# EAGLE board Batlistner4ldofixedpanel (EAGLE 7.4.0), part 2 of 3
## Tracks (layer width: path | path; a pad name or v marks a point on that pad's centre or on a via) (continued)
GND  (via drill 0.5) (continued)
  Top 0.406: IC1.3 15.24,18.73 15.88,17.78 15.88,17.24 C8.2 | 12.06,34.61 v11.75,34.92 12.38,34.29 C16.2 12.97,33.66 C4.2 | IC3.2 41.27,11.74 C13.1 | R12.1 32.06,20.64 v31.11,19.68 30.32,19.05 | v18.41,36.51 18.41,36.2 19.37,35.24 | v23.02,4.29 23.02,3.81 22.7,3.49
  Bottom 0.254: 45.75,9 46.04,8.89 | 9,31.5 SG1.- 8.75,31.75
  other vias: 17.78,12.06 24.13,20.95 12.06,22.23 9.21,27.94 14.29,1.27 31.75,31.11 11.43,38.73 10.16,49.21 34.29,34.92 23.5,30.16 41.91,34.92 44.45,34.92 46.67,39.69 37.78,25.72 20,42.55 1.91,54.61 9.53,54.61 17.14,54.61 22.23,54.61 10.16,46.35 10.16,43.81 1.91,38.73 9.53,1.27 18.1,25.72 24.13,16.67 40.01,1.27 47.62,1.27 60.33,1.27 62.87,6.35 62.87,13.97 62.87,21.59 62.87,33.02 62.87,40.64 62.87,48.26 31.11,54.61 31.91,25.72 40.01,16.51 46.35,20.32 45.88,10.32 53.66,26.04 49.21,29.84 41.91,47.94 38.1,39.37 36.83,42.86 1.91,45.72 14.29,13.02 14.29,7.94 10.17,41.35 21.27,46.99 56.52,43.18
  pour Top: 6.99,-0.64 7.62,19.05 7.94,22.86 7.62,24.77 8.26,35.56 6.99,36.83 0,36.83 0,55.88 64.14,55.88 64.14,31.75 62.23,27.94 64.77,24.13 64.14,0
  pour Bottom: 64.14,0 6.99,-0.64 7.62,15.24 7.62,20 8.26,20.32 8.26,35.56 6.35,37.47 0,36.83 0,55.88 64.77,55.88 64.77,31.75 62.23,27.94 64.77,24.13
GND1  (via drill 0.5)
  Top 0.406: IC7.3 83.82,18.73 84.45,17.78 84.45,17.24 C55.2 | 80.64,34.61 v80.33,34.92 80.96,34.29 C58.2 81.55,33.66 C57.2 | IC9.2 109.86,11.74 C49.1 | R43.1 100.64,20.64 v99.69,19.68 98.9,19.05 | v87,36.51 87,36.2 87.95,35.24 | v91.6,4.29 91.6,3.81 91.28,3.49
  Bottom 0.254: 114.33,9 114.62,8.89 | 77.58,31.5 SG3.- 77.33,31.75
  other vias: 86.36,12.06 92.71,20.95 80.64,22.23 77.79,27.94 82.87,1.27 100.33,31.11 80.01,38.73 78.74,49.21 102.87,34.92 92.08,30.16 110.49,34.92 113.03,34.92 115.25,39.69 106.36,25.72 88.58,42.55 70.48,54.61 78.11,54.61 85.72,54.61 90.81,54.61 78.74,46.35 78.74,43.81 70.48,38.73 78.11,1.27 86.68,25.72 92.71,16.67 108.58,1.27 116.2,1.27 128.91,1.27 131.44,6.35 131.44,13.97 131.44,21.59 131.44,33.02 131.44,40.64 131.44,48.26 99.69,54.61 100.49,25.72 108.58,16.51 114.94,20.32 114.46,10.32 122.24,26.04 117.79,29.84 110.49,47.94 106.68,39.37 105.41,42.86 70.48,45.72 82.87,13.02 82.87,7.94 78.75,41.35 89.85,46.99 125.09,43.18
  pour Top: 75.56,-0.64 76.2,19.05 76.52,22.86 76.2,24.77 76.83,35.56 75.56,36.83 68.58,36.83 68.58,55.88 132.72,55.88 132.72,31.75 130.81,27.94 133.35,24.13 132.72,0
  pour Bottom: 132.72,0 75.56,-0.64 76.2,15.24 76.2,20 76.83,20.32 76.83,35.56 74.93,37.47 68.58,36.83 68.58,55.88 133.35,55.88 133.35,31.75 130.81,27.94 133.35,24.13
GND2  (via drill 0.5)
  Top 0.406: IC13.3 152.4,18.73 153.03,17.78 153.03,17.24 C100.2 | 149.22,34.61 v148.91,34.92 149.54,34.29 C103.2 150.13,33.66 C102.2 | IC15.2 178.44,11.74 C94.1 | R82.1 169.22,20.64 v168.28,19.68 167.48,19.05 | v155.57,36.51 155.57,36.2 156.53,35.24 | v160.18,4.29 160.18,3.81 159.86,3.49
  Bottom 0.254: 182.91,9 183.2,8.89 | 146.16,31.5 SG5.- 145.91,31.75
  other vias: 154.94,12.06 161.29,20.95 149.22,22.23 146.37,27.94 151.45,1.27 168.91,31.11 148.59,38.73 147.32,49.21 171.45,34.92 160.66,30.16 179.07,34.92 181.61,34.92 183.83,39.69 174.94,25.72 157.16,42.55 139.06,54.61 146.69,54.61 154.31,54.61 159.38,54.61 147.32,46.35 147.32,43.81 139.06,38.73 146.69,1.27 155.26,25.72 161.29,16.67 177.16,1.27 184.78,1.27 197.49,1.27 200.03,6.35 200.03,13.97 200.03,21.59 200.03,33.02 200.03,40.64 200.03,48.26 168.28,54.61 169.07,25.72 177.16,16.51 183.51,20.32 183.04,10.32 190.82,26.04 186.37,29.84 179.07,47.94 175.26,39.37 173.99,42.86 139.06,45.72 151.45,13.02 151.45,7.94 147.33,41.35 158.43,46.99 193.68,43.18
  pour Top: 144.15,-0.64 144.78,19.05 145.1,22.86 144.78,24.77 145.41,35.56 144.15,36.83 137.16,36.83 137.16,55.88 201.29,55.88 201.29,31.75 199.39,27.94 201.93,24.13 201.29,0
  pour Bottom: 201.29,0 144.15,-0.64 144.78,15.24 144.78,20 145.41,20.32 145.41,35.56 143.51,37.47 137.16,36.83 137.16,55.88 201.93,55.88 201.93,31.75 199.39,27.94 201.93,24.13
GND3  (via drill 0.5)
  Top 0.406: IC19.3 15.24,79.69 15.88,78.74 15.88,78.2 C145.2 | 12.06,95.57 v11.75,95.89 12.38,95.25 C148.2 12.97,94.61 C147.2 | IC21.2 41.27,72.7 C139.1 | R121.1 32.06,81.59 v31.11,80.64 30.32,80.01 | v18.41,97.47 18.41,97.16 19.37,96.2 | v23.02,65.25 23.02,64.77 22.7,64.45
  Bottom 0.254: 45.75,69.96 46.04,69.85 | 9,92.46 SG7.- 8.75,92.71
  other vias: 17.78,73.03 24.13,81.92 12.06,83.19 9.21,88.9 14.29,62.23 31.75,92.08 11.43,99.69 10.16,110.17 34.29,95.89 23.5,91.12 41.91,95.89 44.45,95.89 46.67,100.65 37.78,86.68 20,103.5 1.91,115.57 9.53,115.57 17.14,115.57 22.23,115.57 10.16,107.31 10.16,104.78 1.91,99.69 9.53,62.23 18.1,86.68 24.13,77.63 40.01,62.23 47.62,62.23 60.33,62.23 62.87,67.31 62.87,74.93 62.87,82.55 62.87,93.98 62.87,101.6 62.87,109.22 31.11,115.57 31.91,86.68 40.01,77.47 46.35,81.28 45.88,71.28 53.66,87 49.21,90.81 41.91,108.9 38.1,100.33 36.83,103.82 1.91,106.68 14.29,73.98 14.29,68.9 10.17,102.31 21.27,107.95 56.52,104.14
  pour Top: 6.99,60.33 7.62,80.01 7.94,83.82 7.62,85.72 8.26,96.52 6.99,97.79 0,97.79 0,116.84 64.14,116.84 64.14,92.71 62.23,88.9 64.77,85.09 64.14,60.96
  pour Bottom: 64.14,60.96 6.99,60.33 7.62,76.2 7.62,80.96 8.26,81.28 8.26,96.52 6.35,98.42 0,97.79 0,116.84 64.77,116.84 64.77,92.71 62.23,88.9 64.77,85.09
GND4  (via drill 0.5)
  Top 0.406: IC25.3 83.82,79.69 84.45,78.74 84.45,78.2 C190.2 | 80.64,95.57 v80.33,95.89 80.96,95.25 C193.2 81.55,94.61 C192.2 | IC27.2 109.86,72.7 C184.1 | R160.1 100.64,81.59 v99.69,80.64 98.9,80.01 | v87,97.47 87,97.16 87.95,96.2 | v91.6,65.25 91.6,64.77 91.28,64.45
  Bottom 0.254: 114.33,69.96 114.62,69.85 | 77.58,92.46 SG9.- 77.33,92.71
  other vias: 86.36,73.03 92.71,81.92 80.64,83.19 77.79,88.9 82.87,62.23 100.33,92.08 80.01,99.69 78.74,110.17 102.87,95.89 92.08,91.12 110.49,95.89 113.03,95.89 115.25,100.65 106.36,86.68 88.58,103.5 70.48,115.57 78.11,115.57 85.72,115.57 90.81,115.57 78.74,107.31 78.74,104.78 70.48,99.69 78.11,62.23 86.68,86.68 92.71,77.63 108.58,62.23 116.2,62.23 128.91,62.23 131.44,67.31 131.44,74.93 131.44,82.55 131.44,93.98 131.44,101.6 131.44,109.22 99.69,115.57 100.49,86.68 108.58,77.47 114.94,81.28 114.46,71.28 122.24,87 117.79,90.81 110.49,108.9 106.68,100.33 105.41,103.82 70.48,106.68 82.87,73.98 82.87,68.9 78.75,102.31 89.85,107.95 125.09,104.14
  pour Top: 75.56,60.33 76.2,80.01 76.52,83.82 76.2,85.72 76.83,96.52 75.56,97.79 68.58,97.79 68.58,116.84 132.72,116.84 132.72,92.71 130.81,88.9 133.35,85.09 132.72,60.96
  pour Bottom: 132.72,60.96 75.56,60.33 76.2,76.2 76.2,80.96 76.83,81.28 76.83,96.52 74.93,98.42 68.58,97.79 68.58,116.84 133.35,116.84 133.35,92.71 130.81,88.9 133.35,85.09
GND5  (via drill 0.5)
  Top 0.406: IC31.3 152.4,79.69 153.03,78.74 153.03,78.2 C235.2 | 149.22,95.57 v148.91,95.89 149.54,95.25 C238.2 150.13,94.61 C237.2 | IC33.2 178.44,72.7 C229.1 | R199.1 169.22,81.59 v168.28,80.64 167.48,80.01 | v155.57,97.47 155.57,97.16 156.53,96.2 | v160.18,65.25 160.18,64.77 159.86,64.45
  Bottom 0.254: 182.91,69.96 183.2,69.85 | 146.16,92.46 SG11.- 145.91,92.71
  other vias: 154.94,73.03 161.29,81.92 149.22,83.19 146.37,88.9 151.45,62.23 168.91,92.08 148.59,99.69 147.32,110.17 171.45,95.89 160.66,91.12 179.07,95.89 181.61,95.89 183.83,100.65 174.94,86.68 157.16,103.5 139.06,115.57 146.69,115.57 154.31,115.57 159.38,115.57 147.32,107.31 147.32,104.78 139.06,99.69 146.69,62.23 155.26,86.68 161.29,77.63 177.16,62.23 184.78,62.23 197.49,62.23 200.03,67.31 200.03,74.93 200.03,82.55 200.03,93.98 200.03,101.6 200.03,109.22 168.28,115.57 169.07,86.68 177.16,77.47 183.51,81.28 183.04,71.28 190.82,87 186.37,90.81 179.07,108.9 175.26,100.33 173.99,103.82 139.06,106.68 151.45,73.98 151.45,68.9 147.33,102.31 158.43,107.95 193.68,104.14
  pour Top: 144.15,60.33 144.78,80.01 145.1,83.82 144.78,85.72 145.41,96.52 144.15,97.79 137.16,97.79 137.16,116.84 201.29,116.84 201.29,92.71 199.39,88.9 201.93,85.09 201.29,60.96
  pour Bottom: 201.29,60.96 144.15,60.33 144.78,76.2 144.78,80.96 145.41,81.28 145.41,96.52 143.51,98.42 137.16,97.79 137.16,116.84 201.93,116.84 201.93,92.71 199.39,88.9 201.93,85.09
N$1  (1 unrouted)
  Top 0.406: C36.2 C35.2 C34.2 C33.2 | C37.2 C38.2 C39.2 C40.2 C3.2 52.7,13.81 | 52.7,13.81 52.71,13.81 C32.2 | 52.7,13.81 52.7,13.34 48.74,13.34 47.78,12.38 47.78,10 48.26,9.53 49.66,9.53 U$1.P$4 50.3,9.39 53.98,5.71 56.66,5.71 U$1.P$3
N$2
  Top 0.406: C14.1 46.35,6.67 R14.1
N$3
  Top 0.254: Q1.C 20.64,1.91 20.32,1.59
  Top 0.406: R5.1 20.32,1.59 C7.1 | R4.2 Q1.C
N$4
  Top 0.406: IC3.7 41.27,17.78 41.91,17.14 44.77,17.14 C15.2
N$5
  Top 0.406: IC1.4 16.51,19.68 18.41,17.78 18.73,17.78 R8.1
N$6
  Top 0.406: R8.2 C9.1
N$7  (1 unrouted)
  Top 0.406: C81.2 C80.2 C79.2 C78.2 | C82.2 C83.2 C84.2 C85.2 C76.2 121.28,13.81 | 121.28,13.81 121.29,13.81 C77.2 | 121.28,13.81 121.28,13.34 117.32,13.34 116.36,12.38 116.36,10 116.84,9.53 118.23,9.53 U$2.P$4 118.88,9.39 122.56,5.71 125.25,5.71 U$2.P$3
N$8
  Top 0.406: IC2.3 27.94,18.41 32.7,18.41 R12.2 34.75,18.73 R13.2 36.66,18.56 R11.1
N$9
  Top 0.406: S1.3 49.39,50.94 50.16,50.16 53.34,50.16 54.61,48.9 D1.A 55.49,47.62 C45.1 C44.1
N$10
  Top 0.406: SG1.+ 9.21,23.81 10.16,22.86 C5.2
N$11
  Top 0.406: 12.06,15.72 Q2.B 11.91,15.88 11.11,15.88 10.79,16.2 R1.1 9.84,15.88 8.89,17.14 8.89,19.37 9.53,20 C5.1
N$12
  Top 0.254: 14.44,15.09 13.02,16.51 11.75,16.51
  Top 0.406: R36.2 14.93,6.67 C6.2 15.88,8.57 16.83,9.53 16.83,10.62 Q3.C 16.66,13.51 R2.2 15.38,13.65 Q2.C 14.44,15.09 | 11.75,16.51 11.43,16.83 11.43,17.78 11.11,18.1 R1.2
N$13
  Top 0.406: 22.22,15.24 R3.2 | C26.1 C25.1 C24.1 C2.1 22.23,12.7 | 22.23,12.7 R3.2 | R2.1 17.14,15.56 R3.2 | R3.2 | 20.95,10.16 R4.1 21.27,9.84 22.23,10.79 22.23,12.7 | 20.95,11.43 22.23,12.7
N$14
  Top 0.406: C7.2 22.86,2.54 24.13,3.81 24.13,5.88 R7.1
N$15
  Top 0.406: R10.1 31.43,11.72 R17.P$1
N$16
  Top 0.406: R6.1 18.1,3.81 | R5.2 17.46,3.81 R6.1 | Q1.B 18.25,3.66 R6.1
N$17
  Top 0.406: C6.1 R6.2
N$18  (via drill 0.5)
  Top 0.406: IC1.1 v12.7,17.78 | v25.72,9.21 23.5,9.21 R7.2
  Bottom 0.406: v12.7,17.78 14.61,17.78 v25.72,9.21
N$19
  Top 0.406: C8.1 14.29,18.09 13.97,18.41 IC1.2
N$20  (via drill 0.5)
  Top 0.406: v21.59,24.13 19.37,24.13 C9.2
  Bottom 0.406: R18.P$3 37.34,44.57 40.01,41.91 40.01,32.38 31.75,24.13 v21.59,24.13
N$21
  Top 0.406: C50.1 114.93,6.67 R45.1
N$22  (via drill 0.5)
  Top 0.406: v43.18,8.89 43.18,12.38 C13.2 42.86,13.65 42.55,13.97 IC3.3
  Bottom 0.406: R18.P$1 31.23,44.57 33.02,46.35 37.47,46.35 43.18,40.64 v43.18,8.89
N$23
  Top 0.406: IC4.9 31.43,26.99 31.75,26.67 33.97,26.67 34.61,27.3 34.61,30.16 R29.2 35.88,30.48 36.83,30.48 36.52,30.16 R31.1 36.88,30.11 C22.2
N$24  (via drill 0.5)  (1 unrouted)
  Top 0.406: IC4.19 v22.54,36.2 | v16.83,48.9 16.83,49.21 17.46,49.85 17.46,51.12
  Bottom 0.406: SCK.TP 22.86,36.2 v22.54,36.2 20.64,36.2 16.83,40.01 v16.83,48.9
N$25  (via drill 0.5)  (1 unrouted)
  Top 0.406: R19.1 v18.73,48.89 | v23.5,39.69 23.81,39.37 IC4.18
  Bottom 0.406: MISO.TP 27.3,36.2 25.4,38.1 23.5,38.1 | 23.5,38.1 20.32,38.1 17.78,40.64 17.78,48.9 v18.73,48.9 | 23.5,38.1 v23.5,39.69
N$26  (via drill 0.5)
  Top 0.406: R20.1 17.46,37.47 17.46,35.88 19.05,34.29 24.45,34.29 25.08,34.92 IC4.17 v25.08,39.37 | v29.84,35.56 29.84,31.11 28.89,30.16 v26.04,30.16
  Bottom 0.406: v25.08,39.37 26.04,39.37 v29.84,35.56 | v26.04,30.16 25.72,30.16 24.77,31.11 MOSI.TP
N$27
  Top 0.406: C23.1 43.18,6.99 C14.2 44.13,7.3 44.45,7.62 44.45,11.43 45.08,12.06 45.09,12.06 47.94,14.92 47.94,19.05 | 47.94,19.05 47.94,22.54 50.16,24.77 52.7,24.77 52.7,23.81 | 52.7,23.81 55.24,23.81 55.56,23.5 55.56,19.05 C36.1 C35.1 C34.1 C33.1 C32.1 | C3.1 C40.1 C39.1 C38.1 C37.1 49.85,23.5 50.16,23.81 52.7,23.81 | IC3.5 47.88,19.11 47.94,19.05
N$28
  Top 0.406: IC2.2 26.67,14.29 C12.2 26.99,11.53 R17.P$3
N$29
  Top 0.406: R21.1 16,36.07 18.41,33.66 25.4,33.66 26.35,34.61 IC4.16
N$30  (via drill 0.5)
  Top 0.406: IC1.6 15.24,23.5 v15.88,22.86 | 35.88,24.29 28.1,24.29 27.3,23.5 24.77,23.5 24.13,22.86 v23.5,22.86 | C11.2 35.88,25.4 35.88,24.29 | 35.88,24.29 C10.2
  Bottom 0.406: v15.88,22.86 v23.5,22.86
N$31
  Top 0.406: R22.1 25.08,41.27 27.62,38.73 IC4.15
N$32
  Top 0.406: C11.1 37.15,27.94 38.42,28.26 R9.2
N$33
  Top 0.406: IC4.14 28.89,39.05 24.57,43.37 R23.1
N$34  (via drill 0.5)
  Top 0.406: R24.1 v20,43.81 | v30.16,39.69 IC4.13
  Bottom 0.406: v20,43.81 24.13,43.81 26.04,41.91 27.94,41.91 v30.16,39.69
N$35  (1 unrouted)
  Top 0.406: IC4.12 31.43,40.96 31.11,41.27 30.96,41.43 30.48,41.91
N$36
  Top 0.406: R15.2 15.56,50.8 IC5.5
N$37
  Top 0.406: IC5.4 15.88,46.35 R19.2
N$38
  Top 0.406: IC5.10 9.53,38.73 10.79,40.01 15.55,40.01 R20.2
N$39
  Top 0.406: IC5.1 13.65,36.39 R21.2
N$40
  Top 0.406: IC5.2 R22.2
N$41
  Top 0.406: IC5.3 14.29,43.81 15.56,45.09 20.83,45.09 R23.2
N$42
  Top 0.406: IC5.8 7.3,43.81 8.57,42.55 15.24,42.55 R24.2
N$43
  Top 0.406: IC5.7 7.94,46.35 9.21,45.09 14.61,45.09 15.24,45.72 21.27,45.72 22.07,44.93 25.56,44.93 25.72,44.77 25.72,43.66 27.78,41.59 R25.2
N$44  (via drill 0.5)
  Top 0.406: v28.26,26.99 R39.2
  Bottom 0.406: IC5.9 7.3,41.27 8.26,40.32 8.26,37.47 10.16,35.56 10.16,34.29 12.06,32.38 12.06,29.84 14.92,26.99 v28.26,26.99
N$45  (via drill 0.5)
  Top 0.406: R40.2 20.48,25.24 18.41,27.3 15.88,27.3 v14.61,28.57
  Bottom 0.406: v14.61,28.57 14.61,33.66 8.89,39.37 8.89,47.62 7.62,48.9 IC5.6
N$46
  Top 0.406: IC4.6 27.62,27.62 25.88,25.88 25.88,25.56 R40.1
N$47
  Top 0.406: C16.1 12.75,31.07 13.34,30.48 14.26,30.48 X1.3 14.32,30.12 16.19,28.26 18.73,28.26 20.32,26.67 25.4,26.67 26.35,27.62 IC4.5
N$48
  Top 0.406: R33.2 42.23,25.98 C21.1
N$49  (via drill 0.5)
  Top 0.406: IC4.20 21.27,39.05 21.59,39.37 v21.59,39.69 C17.2 | v38.1,41.27 39.37,41.27 39.49,41.16 | R29.1 34.92,31.75 v31.75,34.92 | R26.1 40.64,40.01 39.49,41.16 | C18.1 41.27,41.91 | 41.27,41.91 40.24,41.91 39.49,41.16 | 39.49,41.16 | IC6.3 41.27,43.58 41.27,41.91
  Bottom 0.406: v38.1,41.27 33.66,41.27 31.75,39.37 31.75,37.47 | VCC.TP 28.57,31.75 v31.75,34.92 31.75,37.47 | 31.75,37.47 30.48,37.47 26.67,41.27 21.59,41.27 v21.59,39.69
N$50
  Top 0.406: R32.1 39.69,7.94 C23.2
N$51
  Top 0.406: R28.1 47.62,36.2 46.35,37.47 44.34,37.47 C20.1 40.82,37.61 R26.2 40.32,37.46 R27.1
N$52
  Top 0.406: C21.2 42.55,29.7 Q4.B R28.2
N$53
  Top 0.406: Q4.C 39.64,32.38 C22.1 39.37,33.66 38.42,34.61 R27.2
N$54  (via drill 0.5)
  Top 0.406: IC4.1 21.01,28.52 v19.05,30.48
  Bottom 0.406: v19.05,30.48 19.05,33.02 20.32,34.29 RES.TP
N$55
  Top 0.406: C41.1 C19.1 43.81,46.09 | 43.81,46.09 39.85,46.09 IC6.2@1 | R30.2 43.81,48.26 43.81,46.09
N$56
  Top 0.406: IC3.1 38.36,13.91 | 38.36,13.91 R32.2 | 38.36,13.91 38.36,14.55 C43.1
N$57
  Top 0.406: R30.1 R35.2 49.85,47.94 50.8,46.99 C28.1
N$58
  Top 0.406: SG2.+ 9.21,12.7 9.84,12.06 C42.2
N$59  (via drill 0.5)
  Top 0.406: C27.2 R34.1 47.31,25.4 44.13,22.23 v40.64,22.23 | 26.67,19.68 24.13,19.68 22.23,17.78 R3.1 v22.23,20.32 | 26.67,19.68 29.53,19.68 31.11,21.11 31.11,21.59 31.75,22.23 v34.29,22.23 34.92,21.59 R13.1 | IC2.7 26.67,19.68 | IC1.8 12.7,22.86 13.34,22.23 v13.97,22.23
  Bottom 0.406: v34.29,22.23 36.2,24.13 38.73,24.13 v40.64,22.23 | v13.97,22.23 14.61,22.23 15.24,21.59 20.95,21.59 v22.23,20.32
N$60
  Top 0.406: R36.1 C42.1 12.88,10.16 Q3.B
N$61
  Top 0.406: C43.2 R37.1
N$62
  Top 0.406: R37.2 38.41,16.82 40.01,18.41 IC3.8
N$63
  Top 0.406: C4.1 15.88,33.66 15.88,31.75 | 15.88,31.75 15.88,29.84 16.51,29.21 18.73,29.21 20.64,27.3 24.77,27.3 25.08,27.62 IC4.4 | X1.1 15.94,31.82 15.88,31.75
N$64
  Top 0.406: U$1.P$1 59.37,4.26 R38.2
N$65
  Top 0.406: U$1.P$5 50.01,11.28 50.32,11.59 53.17,11.6 53.98,10.79 56.48,10.79 U$1.P$6 57.45,11.1 SP1.+
N$66
  Top 0.406: R39.1 30.16,26.51 28.89,27.78 IC4.7
N$67
  Top 0.406: S1.2 52.53,52.88 55.24,50.16 57.15,50.16 57.78,49.53 60.33,49.53 60.96,48.9 60.96,43.18 G1.+
N$68
  Top 0.406: IC9.7 109.86,17.78 110.49,17.14 113.34,17.14 C51.2
N$69
  Top 0.406: IC7.4 85.09,19.68 87,17.78 87.31,17.78 R54.1
N$70
  Top 0.406: R54.2 C56.1
N$71
  Top 0.406: SG3.+ 77.79,23.81 78.74,22.86 C52.2
N$72
  Top 0.406: 80.64,15.72 Q6.B 80.5,15.88 79.69,15.88 79.37,16.2 R16.1 78.42,15.88 77.47,17.14 77.47,19.37 78.11,20 C52.1
N$73
  Top 0.254: 83.02,15.09 81.6,16.51 80.33,16.51
  Top 0.406: R74.2 83.51,6.67 C53.2 84.46,8.57 85.41,9.53 85.41,10.62 Q8.C 85.24,13.51 R48.2 83.97,13.65 Q6.C 83.02,15.09 | 80.33,16.51 80.01,16.83 80.01,17.78 79.69,18.1 R16.2
N$74
  Top 0.406: 90.8,15.24 R49.2 | C69.1 C68.1 C67.1 C66.1 90.81,12.7 | 90.81,12.7 R49.2 | R48.1 85.72,15.56 R49.2 | R49.2 | 89.53,10.16 R50.1 89.85,9.84 90.81,10.79 90.81,12.7 | 89.53,11.43 90.81,12.7
N$75
  Top 0.406: R52.1 86.68,3.81 | R51.2 86.05,3.81 R52.1 | Q5.B 86.83,3.66 R52.1
N$76
  Top 0.406: C53.1 R52.2
N$77
  Top 0.254: Q5.C 89.22,1.91 88.9,1.59
  Top 0.406: R51.1 88.9,1.59 C54.1 | R50.2 Q5.C
N$78
  Top 0.406: C54.2 91.44,2.54 92.71,3.81 92.71,5.88 R53.1
N$79  (via drill 0.5)
  Top 0.406: IC7.1 v81.28,17.78 | v94.3,9.21 92.08,9.21 R53.2
  Bottom 0.406: v81.28,17.78 83.19,17.78 v94.3,9.21
N$80
  Top 0.406: C55.1 82.87,18.09 82.55,18.41 IC7.2
N$81  (via drill 0.5)
  Top 0.406: v90.17,24.13 87.95,24.13 C56.2
  Bottom 0.406: R47.P$3 105.92,44.57 108.58,41.91 108.58,32.38 100.33,24.13 v90.17,24.13
N$82  (via drill 0.5)
  Top 0.406: v111.76,8.89 111.76,12.38 C49.2 111.44,13.65 111.12,13.97 IC9.3
  Bottom 0.406: R47.P$1 99.81,44.57 101.6,46.35 106.05,46.35 111.76,40.64 v111.76,8.89
N$83
  Top 0.406: C65.1 111.76,6.99 C50.2 112.71,7.3 113.03,7.62 113.03,11.43 113.66,12.06 113.67,12.06 116.52,14.92 116.52,19.05 | 116.52,19.05 116.52,22.54 118.75,24.77 121.28,24.77 121.28,23.81 | 121.28,23.81 123.83,23.81 124.14,23.5 124.14,19.05 C81.1 C80.1 C79.1 C78.1 C77.1 | C76.1 C85.1 C84.1 C83.1 C82.1 118.43,23.5 118.75,23.81 121.28,23.81 | IC9.5 116.46,19.11 116.52,19.05
N$84
  Top 0.406: IC8.3 96.52,18.41 101.28,18.41 R43.2 103.33,18.73 R44.2 105.23,18.56 R42.1
N$85
  Top 0.406: IC8.2 95.25,14.29 C48.2 95.57,11.53 R46.P$3
N$86  (via drill 0.5)
  Top 0.406: IC7.6 83.82,23.5 v84.45,22.86 | 104.46,24.29 96.68,24.29 95.89,23.5 93.34,23.5 92.71,22.86 v92.08,22.86 | C47.2 104.46,25.4 104.46,24.29 | 104.46,24.29 C46.2
  Bottom 0.406: v84.45,22.86 v92.08,22.86
N$87
  Top 0.406: C47.1 105.72,27.94 107,28.26 R55.2
N$88
  Top 0.406: R41.1 100.02,11.72 R46.P$1
N$89  (via drill 0.5)  (1 unrouted)
  Top 0.406: IC10.19 v91.12,36.2 | v85.41,48.9 85.41,49.21 86.04,49.85 86.04,51.12
  Bottom 0.406: SCK1.TP 91.44,36.2 v91.12,36.2 89.22,36.2 85.41,40.01 v85.41,48.9
N$90  (via drill 0.5)  (1 unrouted)
  Top 0.406: R57.1 v87.31,48.89 | v92.08,39.69 92.39,39.37 IC10.18
  Bottom 0.406: MISO1.TP 95.89,36.2 93.98,38.1 92.08,38.1 | 92.08,38.1 88.9,38.1 86.36,40.64 86.36,48.9 v87.31,48.9 | 92.08,38.1 v92.08,39.69
N$91  (via drill 0.5)
  Top 0.406: R58.1 86.04,37.47 86.04,35.88 87.63,34.29 93.03,34.29 93.66,34.92 IC10.17 v93.66,39.37 | v98.42,35.56 98.42,31.11 97.47,30.16 v94.61,30.16
  Bottom 0.406: v93.66,39.37 94.61,39.37 v98.42,35.56 | v94.61,30.16 94.3,30.16 93.34,31.11 MOSI1.TP
N$92
  Top 0.406: R59.1 84.58,36.07 87,33.66 93.98,33.66 94.93,34.61 IC10.16
N$93
  Top 0.406: R60.1 93.66,41.27 96.2,38.73 IC10.15
N$94
  Top 0.406: IC10.14 97.47,39.05 93.15,43.37 R61.1
N$95  (via drill 0.5)
  Top 0.406: R62.1 v88.58,43.81 | v98.74,39.69 IC10.13
  Bottom 0.406: v88.58,43.81 92.71,43.81 94.61,41.91 96.52,41.91 v98.74,39.69
N$96  (1 unrouted)
  Top 0.406: IC10.12 100.01,40.96 99.69,41.27 99.54,41.43 99.06,41.91
N$97
  Top 0.406: R56.2 84.14,50.8 IC11.5
N$98
  Top 0.406: IC11.4 84.46,46.35 R57.2
N$99
  Top 0.406: IC11.10 78.11,38.73 79.38,40.01 84.14,40.01 R58.2
N$100
  Top 0.406: IC11.1 82.23,36.39 R59.2
N$101
  Top 0.406: IC11.2 R60.2
N$102
  Top 0.406: IC11.3 82.87,43.81 84.14,45.09 89.41,45.09 R61.2
N$103
  Top 0.406: IC11.8 75.88,43.81 77.15,42.55 83.82,42.55 R62.2
N$104
  Top 0.406: IC11.7 76.52,46.35 77.79,45.09 83.19,45.09 83.82,45.72 89.85,45.72 90.65,44.93 94.14,44.93 94.3,44.77 94.3,43.66 96.36,41.59 R63.2
N$105  (via drill 0.5)
  Top 0.406: v96.84,26.99 R77.2
  Bottom 0.406: IC11.9 75.88,41.27 76.83,40.32 76.83,37.47 78.74,35.56 78.74,34.29 80.64,32.38 80.64,29.84 83.5,26.99 v96.84,26.99
N$106  (via drill 0.5)
  Top 0.406: R78.2 89.06,25.24 87,27.3 84.45,27.3 v83.19,28.57
  Bottom 0.406: v83.19,28.57 83.19,33.66 77.47,39.37 77.47,47.62 76.2,48.9 IC11.6
N$107
  Top 0.406: C58.1 81.33,31.07 81.92,30.48 82.84,30.48 X2.3 82.91,30.12 84.77,28.26 87.31,28.26 88.9,26.67 93.98,26.67 94.93,27.62 IC10.5
N$108  (via drill 0.5)
  Top 0.406: IC10.20 89.85,39.05 90.17,39.37 v90.17,39.69 C59.2 | v106.68,41.27 107.95,41.27 108.07,41.16 | R68.1 103.5,31.75 v100.33,34.92 | R64.1 109.22,40.01 108.07,41.16 | C60.1 109.86,41.91 | 109.86,41.91 108.82,41.91 108.07,41.16 | 108.07,41.16 | IC12.3 109.86,43.58 109.86,41.91
  Bottom 0.406: v106.68,41.27 102.23,41.27 100.33,39.37 100.33,37.47 | VCC1.TP 97.16,31.75 v100.33,34.92 100.33,37.47 | 100.33,37.47 99.06,37.47 95.25,41.27 90.17,41.27 v90.17,39.69
N$109
  Top 0.406: R66.1 116.2,36.2 114.94,37.47 112.92,37.47 C62.1 109.4,37.61 R64.2 108.9,37.46 R65.1
N$110
  Top 0.406: C63.2 111.12,29.7 Q7.B R66.2
N$111
  Top 0.406: Q7.C 108.22,32.38 C64.1 107.95,33.66 107,34.61 R65.2
N$112
  Top 0.406: C86.1 C61.1 112.39,46.09 | 112.39,46.09 108.43,46.09 IC12.2@1 | R67.2 112.39,48.26 112.39,46.09
N$113  (via drill 0.5)
  Top 0.406: IC10.1 89.59,28.52 v87.63,30.48
  Bottom 0.406: v87.63,30.48 87.63,33.02 88.9,34.29 RES1.TP
N$114
  Top 0.406: IC10.9 100.01,26.99 100.33,26.67 102.55,26.67 103.19,27.3 103.19,30.16 R68.2 104.46,30.48 105.41,30.48 105.09,30.16 R69.1 105.46,30.11 C64.2
N$115
  Top 0.406: R70.1 108.27,7.94 C65.2
N$116
  Top 0.406: IC9.1 106.94,13.91 | 106.94,13.91 R70.2 | 106.94,13.91 106.94,14.55 C88.1
N$117
  Top 0.406: R71.2 110.81,25.98 C63.1
N$118  (via drill 0.5)
  Top 0.406: C70.2 R72.1 115.89,25.4 112.71,22.23 v109.22,22.23 | 95.25,19.68 92.71,19.68 90.81,17.78 R49.1 v90.81,20.32 | 95.25,19.68 98.11,19.68 99.69,21.11 99.69,21.59 100.33,22.23 v102.87,22.23 103.5,21.59 R44.1 | IC8.7 95.25,19.68 | IC7.8 81.28,22.86 81.92,22.23 v82.55,22.23
  Bottom 0.406: v102.87,22.23 104.78,24.13 107.31,24.13 v109.22,22.23 | v82.55,22.23 83.19,22.23 83.82,21.59 89.53,21.59 v90.81,20.32
N$119
  Top 0.406: R67.1 R73.2 118.43,47.94 119.38,46.99 C71.1
N$120
  Top 0.406: SG4.+ 77.79,12.7 78.42,12.06 C87.2
N$121
  Top 0.406: R74.1 C87.1 81.45,10.16 Q8.B
N$122
  Top 0.406: C88.2 R75.1
N$123
  Top 0.406: R75.2 107,16.82 108.58,18.41 IC9.8
N$124
  Top 0.406: U$2.P$1 127.95,4.26 R76.2
N$125
  Top 0.406: U$2.P$5 118.59,11.28 118.9,11.59 121.75,11.6 122.56,10.79 125.06,10.79 U$2.P$6 126.03,11.1 SP2.+
N$126
  Top 0.406: C57.1 84.45,33.66 84.45,31.75 | 84.45,31.75 84.45,29.84 85.09,29.21 87.31,29.21 89.22,27.3 93.34,27.3 93.66,27.62 IC10.4 | X2.1 84.52,31.82 84.45,31.75
N$127
  Top 0.406: IC10.6 96.2,27.62 94.46,25.88 94.46,25.56 R78.1
N$128
  Top 0.406: R77.1 98.74,26.51 97.47,27.78 IC10.7
N$129
  Top 0.406: S2.3 117.97,50.94 118.75,50.16 121.92,50.16 123.19,48.9 D2.A 124.07,47.62 C90.1 C89.1
N$130
  Top 0.406: S2.2 121.11,52.88 123.83,50.16 125.73,50.16 126.36,49.53 128.91,49.53 129.54,48.9 129.54,43.18 G2.+
N$131  (1 unrouted)
  Top 0.406: C126.2 C125.2 C124.2 C123.2 | C127.2 C128.2 C129.2 C130.2 C121.2 189.87,13.81 | 189.87,13.81 C122.2 | 189.87,13.81 189.87,13.34 185.9,13.34 184.94,12.38 184.94,10 185.42,9.53 186.81,9.53 U$3.P$4 187.46,9.39 191.13,5.71 193.82,5.71 U$3.P$3
N$132
  Top 0.406: C95.1 183.51,6.67 R84.1
N$133
  Top 0.406: IC15.7 178.44,17.78 179.07,17.14 181.93,17.14 C96.2
N$134
  Top 0.406: IC13.4 153.67,19.68 155.57,17.78 155.89,17.78 R93.1
N$135
  Top 0.406: R93.2 C101.1
N$136
  Top 0.406: SG5.+ 146.37,23.81 147.32,22.86 C97.2
N$137
  Top 0.406: 149.22,15.72 Q10.B 149.07,15.88 148.27,15.88 147.95,16.2 R79.1 147,15.88 146.05,17.14 146.05,19.37 146.69,20 C97.1
N$138
  Top 0.254: 151.59,15.09 150.18,16.51 148.91,16.51
  Top 0.406: R113.2 152.09,6.67 C98.2 153.04,8.57 153.99,9.53 153.99,10.62 Q12.C 153.82,13.51 R87.2 152.54,13.65 Q10.C 151.59,15.09 | 148.91,16.51 148.59,16.83 148.59,17.78 148.27,18.1 R79.2
N$139
  Top 0.406: 159.38,15.24 R88.2 | C114.1 C113.1 C112.1 C111.1 159.38,12.7 | 159.38,12.7 R88.2 | R87.1 154.3,15.56 R88.2 | R88.2 | 158.12,10.16 R89.1 158.43,9.84 159.38,10.79 159.38,12.7 | 158.12,11.43 159.38,12.7
N$140
  Top 0.406: R91.1 155.26,3.81 | R90.2 154.62,3.81 R91.1 | Q9.B 155.41,3.66 R91.1
N$141
  Top 0.406: C98.1 R91.2
N$142
  Top 0.254: Q9.C 157.8,1.91 157.48,1.59
  Top 0.406: R90.1 157.48,1.59 C99.1 | R89.2 Q9.C
N$143
  Top 0.406: C99.2 160.02,2.54 161.29,3.81 161.29,5.88 R92.1
N$144  (via drill 0.5)
  Top 0.406: IC13.1 v149.86,17.78 | v162.88,9.21 160.66,9.21 R92.2
  Bottom 0.406: v149.86,17.78 151.76,17.78 v162.88,9.21
N$145
  Top 0.406: C100.1 151.45,18.09 151.13,18.41 IC13.2
N$146  (via drill 0.5)
  Top 0.406: v158.75,24.13 156.53,24.13 C101.2
  Bottom 0.406: R86.P$3 174.5,44.57 177.16,41.91 177.16,32.38 168.91,24.13 v158.75,24.13
N$147  (via drill 0.5)
  Top 0.406: v180.34,8.89 180.34,12.38 C94.2 180.02,13.65 179.71,13.97 IC15.3
  Bottom 0.406: R86.P$1 168.4,44.57 170.18,46.35 174.62,46.35 180.34,40.64 v180.34,8.89
N$148
  Top 0.406: C110.1 180.34,6.99 C95.2 181.29,7.3 181.61,7.62 181.61,11.43 182.24,12.06 182.25,12.06 185.1,14.92 185.1,19.05 | 185.1,19.05 185.1,22.54 187.32,24.77 189.87,24.77 189.87,23.81 | 189.87,23.81 192.41,23.81 192.72,23.5 192.72,19.05 C126.1 C125.1 C124.1 C123.1 C122.1 | C121.1 C130.1 C129.1 C128.1 C127.1 187.01,23.5 187.32,23.81 189.87,23.81 | IC15.5 185.04,19.11 185.1,19.05
N$149
  Top 0.406: IC14.3 165.1,18.41 169.86,18.41 R82.2 171.91,18.73 R83.2 173.81,18.56 R81.1
N$150
  Top 0.406: IC14.2 163.83,14.29 C93.2 164.15,11.53 R85.P$3
N$151  (via drill 0.5)
  Top 0.406: IC13.6 152.4,23.5 v153.03,22.86 | 173.04,24.29 165.26,24.29 164.47,23.5 161.93,23.5 161.29,22.86 v160.66,22.86 | C92.2 173.04,25.4 173.04,24.29 | 173.04,24.29 C91.2
  Bottom 0.406: v153.03,22.86 v160.66,22.86
N$152
  Top 0.406: C92.1 174.31,27.94 175.58,28.26 R94.2
N$153
  Top 0.406: R80.1 168.59,11.72 R85.P$1
N$154  (via drill 0.5)  (1 unrouted)
  Top 0.406: IC16.19 v159.7,36.2 | v153.99,48.9 153.99,49.21 154.62,49.85 154.62,51.12
  Bottom 0.406: SCK2.TP 160.02,36.2 v159.7,36.2 157.8,36.2 153.99,40.01 v153.99,48.9
N$155  (via drill 0.5)  (1 unrouted)
  Top 0.406: R96.1 v155.89,48.89 | v160.66,39.69 160.97,39.37 IC16.18
  Bottom 0.406: MISO2.TP 164.47,36.2 162.56,38.1 160.66,38.1 | 160.66,38.1 157.48,38.1 154.94,40.64 154.94,48.9 v155.89,48.9 | 160.66,38.1 v160.66,39.69
N$156  (via drill 0.5)
  Top 0.406: R97.1 154.62,37.47 154.62,35.88 156.21,34.29 161.61,34.29 162.24,34.92 IC16.17 v162.24,39.37 | v167,35.56 167,31.11 166.05,30.16 v163.19,30.16
  Bottom 0.406: v162.24,39.37 163.19,39.37 v167,35.56 | v163.19,30.16 162.88,30.16 161.93,31.11 MOSI2.TP
N$157
  Top 0.406: R98.1 153.16,36.07 155.57,33.66 162.56,33.66 163.51,34.61 IC16.16
N$158
  Top 0.406: R99.1 162.24,41.27 164.78,38.73 IC16.15
N$159
  Top 0.406: IC16.14 166.05,39.05 161.73,43.37 R100.1
N$160  (via drill 0.5)
  Top 0.406: R101.1 v157.16,43.81 | v167.32,39.69 IC16.13
  Bottom 0.406: v157.16,43.81 161.29,43.81 163.19,41.91 165.1,41.91 v167.32,39.69
N$161  (1 unrouted)
  Top 0.406: IC16.12 168.59,40.96 168.28,41.27 168.12,41.43 167.64,41.91
N$162
  Top 0.406: R95.2 152.72,50.8 IC17.5
N$163
  Top 0.406: IC17.4 153.04,46.35 R96.2
N$164
  Top 0.406: IC17.10 146.69,38.73 147.96,40.01 152.72,40.01 R97.2
N$165
  Top 0.406: IC17.1 150.81,36.39 R98.2
N$166
  Top 0.406: IC17.2 R99.2
N$167
  Top 0.406: IC17.3 151.45,43.81 152.72,45.09 157.99,45.09 R100.2
N$168
  Top 0.406: IC17.8 144.46,43.81 145.73,42.55 152.4,42.55 R101.2
N$169
  Top 0.406: IC17.7 145.1,46.35 146.37,45.09 151.76,45.09 152.4,45.72 158.43,45.72 159.23,44.93 162.72,44.93 162.88,44.77 162.88,43.66 164.94,41.59 R102.2
N$170  (via drill 0.5)
  Top 0.406: v165.42,26.99 R116.2
  Bottom 0.406: IC17.9 144.46,41.27 145.41,40.32 145.41,37.47 147.32,35.56 147.32,34.29 149.22,32.38 149.22,29.84 152.08,26.99 v165.42,26.99
N$171  (via drill 0.5)
  Top 0.406: R117.2 157.64,25.24 155.57,27.3 153.03,27.3 v151.76,28.57
  Bottom 0.406: v151.76,28.57 151.76,33.66 146.05,39.37 146.05,47.62 144.78,48.9 IC17.6
N$172
  Top 0.406: C103.1 149.91,31.07 150.5,30.48 151.42,30.48 X3.3 151.49,30.12 153.35,28.26 155.89,28.26 157.48,26.67 162.56,26.67 163.51,27.62 IC16.5
N$173  (via drill 0.5)
  Top 0.406: IC16.20 158.43,39.05 158.75,39.37 v158.75,39.69 C104.2 | v175.26,41.27 176.53,41.27 176.65,41.16 | R107.1 172.09,31.75 v168.91,34.92 | R103.1 177.8,40.01 176.65,41.16 | C105.1 178.44,41.91 | 178.44,41.91 177.4,41.91 176.65,41.16 | 176.65,41.16 | IC18.3 178.44,43.58 178.44,41.91
  Bottom 0.406: v175.26,41.27 170.81,41.27 168.91,39.37 168.91,37.47 | VCC2.TP 165.74,31.75 v168.91,34.92 168.91,37.47 | 168.91,37.47 167.64,37.47 163.83,41.27 158.75,41.27 v158.75,39.69
N$174
  Top 0.406: R105.1 184.78,36.2 183.51,37.47 181.5,37.47 C107.1 177.98,37.61 R103.2 177.48,37.46 R104.1
N$175
  Top 0.406: C108.2 179.71,29.7 Q11.B R105.2
N$176
  Top 0.406: Q11.C 176.8,32.38 C109.1 176.53,33.66 175.58,34.61 R104.2
N$177
  Top 0.406: C131.1 C106.1 180.97,46.09 | 180.97,46.09 177.01,46.09 IC18.2@1 | R106.2 180.97,48.26 180.97,46.09
N$178  (via drill 0.5)
  Top 0.406: IC16.1 158.17,28.52 v156.21,30.48
  Bottom 0.406: v156.21,30.48 156.21,33.02 157.48,34.29 RES2.TP
N$179
  Top 0.406: IC16.9 168.59,26.99 168.91,26.67 171.13,26.67 171.77,27.3 171.77,30.16 R107.2 173.04,30.48 173.99,30.48 173.68,30.16 R108.1 174.04,30.11 C109.2
N$180
  Top 0.406: R109.1 176.85,7.94 C110.2
N$181
  Top 0.406: IC15.1 175.52,13.91 | 175.52,13.91 R109.2 | 175.52,13.91 175.52,14.55 C133.1
N$182
  Top 0.406: R110.2 179.38,25.98 C108.1
N$183  (via drill 0.5)
  Top 0.406: C115.2 R111.1 184.47,25.4 181.29,22.23 v177.8,22.23 | 163.83,19.68 161.29,19.68 159.38,17.78 R88.1 v159.38,20.32 | 163.83,19.68 166.69,19.68 168.28,21.11 168.28,21.59 168.91,22.23 v171.45,22.23 172.09,21.59 R83.1 | IC14.7 163.83,19.68 | IC13.8 149.86,22.86 150.5,22.23 v151.13,22.23
  Bottom 0.406: v171.45,22.23 173.35,24.13 175.9,24.13 v177.8,22.23 | v151.13,22.23 151.76,22.23 152.4,21.59 158.12,21.59 v159.38,20.32
N$184
  Top 0.406: R106.1 R112.2 187.01,47.94 187.96,46.99 C116.1
N$185
  Top 0.406: SG6.+ 146.37,12.7 147,12.06 C132.2
N$186
  Top 0.406: R113.1 C132.1 150.03,10.16 Q12.B
N$187
  Top 0.406: C133.2 R114.1
N$188
  Top 0.406: R114.2 175.57,16.82 177.16,18.41 IC15.8
N$189
  Top 0.406: U$3.P$1 196.53,4.26 R115.2
N$190
  Top 0.406: U$3.P$5 187.17,11.28 187.48,11.59 190.34,11.6 191.13,10.79 193.65,10.79 U$3.P$6 194.61,11.1 SP3.+
N$191
  Top 0.406: C102.1 153.03,33.66 153.03,31.75 | 153.03,31.75 153.03,29.84 153.67,29.21 155.89,29.21 157.8,27.3 161.93,27.3 162.24,27.62 IC16.4 | X3.1 153.1,31.82 153.03,31.75
N$192
  Top 0.406: IC16.6 164.78,27.62 163.04,25.88 163.04,25.56 R117.1
N$193
  Top 0.406: R116.1 167.32,26.51 166.05,27.78 IC16.7
N$194
  Top 0.406: S3.3 186.55,50.94 187.32,50.16 190.5,50.16 191.77,48.9 D3.A 192.65,47.62 C135.1 C134.1
N$195
  Top 0.406: S3.2 189.69,52.88 192.41,50.16 194.31,50.16 194.94,49.53 197.49,49.53 198.12,48.9 198.12,43.18 G3.+
N$196  (1 unrouted)
  Top 0.406: C171.2 C170.2 C169.2 C168.2 | C172.2 C173.2 C174.2 C175.2 C166.2 52.7,74.77 | 52.7,74.77 52.71,74.77 C167.2 | 52.7,74.77 52.7,74.3 48.74,74.3 47.78,73.34 47.78,70.96 48.26,70.48 49.66,70.48 U$4.P$4 50.3,70.36 53.98,66.67 56.66,66.67 U$4.P$3
N$197
  Top 0.406: C140.1 46.35,67.63 R123.1
N$198
  Top 0.406: IC21.7 41.27,78.74 41.91,78.11 44.77,78.11 C141.2
N$199
  Top 0.406: IC19.4 16.51,80.64 18.41,78.74 18.73,78.74 R132.1
N$200
  Top 0.406: R132.2 C146.1
N$201
  Top 0.406: SG7.+ 9.21,84.77 10.16,83.82 C142.2
N$202
  Top 0.406: 12.06,76.69 Q14.B 11.91,76.83 11.11,76.83 10.79,77.16 R118.1 9.84,76.84 9.84,76.83 8.89,78.11 8.89,80.33 9.53,80.97 C142.1
N$203
  Top 0.254: 14.44,76.05 13.02,77.47 11.75,77.47
  Top 0.406: R152.2 14.93,67.63 C143.2 15.88,69.53 16.83,70.48 16.83,71.58 Q16.C 16.66,74.47 R126.2 15.38,74.61 Q14.C 14.44,76.05 | 11.75,77.47 11.43,77.79 11.43,78.74 11.11,79.06 R118.2
N$204
  Top 0.406: 22.22,76.2 R127.2 | C159.1 C158.1 C157.1 C156.1 22.23,73.66 | 22.23,73.66 R127.2 | R126.1 17.14,76.52 R127.2 | R127.2 | 20.95,71.12 R128.1 21.27,70.8 22.23,71.75 22.23,73.66 | 20.95,72.39 22.23,73.66
N$205
  Top 0.406: R130.1 18.1,64.77 | R129.2 17.46,64.78 R130.1 | Q13.B 18.25,64.62 R130.1
N$206
  Top 0.406: C143.1 R130.2
N$207
  Top 0.254: Q13.C 20.64,62.87 20.32,62.55
  Top 0.406: R129.1 20.32,62.55 C144.1 | R128.2 Q13.C
N$208
  Top 0.406: C144.2 22.86,63.5 24.13,64.77 24.13,66.84 R131.1
N$209  (via drill 0.5)
  Top 0.406: IC19.1 v12.7,78.74 | v25.72,70.17 23.5,70.17 R131.2
  Bottom 0.406: v12.7,78.74 14.61,78.74 v25.72,70.17
N$210
  Top 0.406: C145.1 14.29,79.06 13.97,79.38 IC19.2
N$211  (via drill 0.5)
  Top 0.406: v21.59,85.09 19.37,85.09 C146.2
  Bottom 0.406: R125.P$3 37.34,105.53 40.01,102.87 40.01,93.34 31.75,85.09 v21.59,85.09
N$212  (via drill 0.5)
  Top 0.406: v43.18,69.85 43.18,73.34 C139.2 42.86,74.61 42.55,74.93 IC21.3
  Bottom 0.406: R125.P$1 31.23,105.53 33.02,107.31 37.47,107.31 43.18,101.6 v43.18,69.85
N$213
  Top 0.406: C155.1 43.18,67.94 C140.2 44.13,68.26 44.45,68.58 44.45,72.39 45.08,73.02 45.09,73.03 47.94,75.88 47.94,80.01 | 47.94,80.01 47.94,83.5 50.16,85.72 52.7,85.72 52.7,84.77 | 52.7,84.77 55.24,84.77 55.56,84.45 55.56,80.01 C171.1 C170.1 C169.1 C168.1 C167.1 | C166.1 C175.1 C174.1 C173.1 C172.1 49.85,84.46 50.16,84.77 52.7,84.77 | IC21.5 47.88,80.07 47.94,80.01
N$214
  Top 0.406: IC20.3 27.94,79.38 32.7,79.38 R121.2 34.75,79.69 R122.2 36.66,79.52 R120.1
N$215
  Top 0.406: IC20.2 26.67,75.25 C138.2 26.99,72.49 R124.P$3
N$216  (via drill 0.5)
  Top 0.406: IC19.6 15.24,84.45 v15.88,83.82 | 35.88,85.25 28.1,85.25 27.3,84.45 24.77,84.45 24.13,83.82 v23.5,83.82 | C137.2 35.88,86.36 35.88,85.25 | 35.88,85.25 C136.2
  Bottom 0.406: v15.88,83.82 v23.5,83.82
N$217
  Top 0.406: C137.1 37.15,88.9 38.42,89.22 R133.2
N$218
  Top 0.406: R119.1 31.43,72.69 R124.P$1
N$219  (via drill 0.5)  (1 unrouted)
  Top 0.406: IC22.19 v22.54,97.16 | v16.83,109.86 16.83,110.17 17.46,110.81 17.46,112.08
  Bottom 0.406: SCK3.TP 22.86,97.16 v22.54,97.16 20.64,97.16 16.83,100.97 v16.83,109.86
N$220  (via drill 0.5)  (1 unrouted)
  Top 0.406: R135.1 v18.73,109.85 | v23.5,100.65 23.81,100.33 IC22.18
  Bottom 0.406: MISO3.TP 27.3,97.16 25.4,99.06 23.5,99.06 | 23.5,99.06 20.32,99.06 17.78,101.6 17.78,109.86 v18.73,109.86 | 23.5,99.06 v23.5,100.65
N$221  (via drill 0.5)
  Top 0.406: R136.1 17.46,98.43 17.46,96.84 19.05,95.25 24.45,95.25 25.08,95.89 IC22.17 v25.08,100.33 | v29.84,96.52 29.84,92.08 28.89,91.12 v26.04,91.12
  Bottom 0.406: v25.08,100.33 26.04,100.33 v29.84,96.52 | v26.04,91.12 25.72,91.12 24.77,92.08 MOSI3.TP
N$222
  Top 0.406: R137.1 16,97.03 18.41,94.61 25.4,94.61 26.35,95.57 IC22.16
N$223
  Top 0.406: R138.1 25.08,102.23 27.62,99.69 IC22.15
N$224
  Top 0.406: IC22.14 28.89,100.01 24.57,104.33 R139.1
N$225  (via drill 0.5)
  Top 0.406: R140.1 v20,104.78 | v30.16,100.65 IC22.13
  Bottom 0.406: v20,104.78 24.13,104.78 26.04,102.87 27.94,102.87 v30.16,100.65
N$226  (1 unrouted)
  Top 0.406: IC22.12 31.43,101.92 31.11,102.23 30.96,102.39 30.48,102.87
N$227
  Top 0.406: R134.2 15.56,111.76 IC23.5
N$228
  Top 0.406: IC23.4 15.88,107.31 R135.2
N$229
  Top 0.406: IC23.10 9.53,99.69 10.79,100.97 15.55,100.97 R136.2
N$230
  Top 0.406: IC23.1 13.65,97.35 R137.2
N$231
  Top 0.406: IC23.2 R138.2
N$232
  Top 0.406: IC23.3 14.29,104.78 15.56,106.05 20.83,106.05 R139.2
N$233
  Top 0.406: IC23.8 7.3,104.78 8.57,103.5 15.24,103.5 R140.2
N$234
  Top 0.406: IC23.7 7.94,107.31 9.21,106.05 14.61,106.05 15.24,106.68 21.27,106.68 22.07,105.89 25.56,105.89 25.72,105.73 25.72,104.62 27.78,102.55 R141.2
N$235  (via drill 0.5)
  Top 0.406: v28.26,87.95 R155.2
  Bottom 0.406: IC23.9 7.3,102.23 8.26,101.28 8.26,98.42 10.16,96.52 10.16,95.25 12.06,93.34 12.06,90.81 14.92,87.95 v28.26,87.95
N$236  (via drill 0.5)
  Top 0.406: R156.2 20.48,86.2 18.41,88.27 15.88,88.27 v14.61,89.53
  Bottom 0.406: v14.61,89.53 14.61,94.61 8.89,100.33 8.89,108.58 7.62,109.86 IC23.6
N$237
  Top 0.406: C148.1 12.75,92.03 13.34,91.44 14.26,91.44 X4.3 14.32,91.08 16.19,89.22 18.73,89.22 20.32,87.63 25.4,87.63 26.35,88.58 IC22.5
N$238  (via drill 0.5)
  Top 0.406: IC22.20 21.27,100.01 21.59,100.33 v21.59,100.65 C149.2 | v38.1,102.23 39.37,102.23 39.49,102.12 | R146.1 34.92,92.71 v31.75,95.89 | R142.1 40.64,100.97 39.49,102.12 | C150.1 41.27,102.87 | 41.27,102.87 40.24,102.87 39.49,102.12 | 39.49,102.12 | IC24.3 41.27,104.54 41.27,102.87
  Bottom 0.406: v38.1,102.23 33.66,102.23 31.75,100.33 31.75,98.42 | VCC3.TP 28.57,92.71 v31.75,95.89 31.75,98.42 | 31.75,98.42 30.48,98.42 26.67,102.23 21.59,102.23 v21.59,100.65
N$239
  Top 0.406: R144.1 47.62,97.16 46.35,98.42 44.34,98.42 C152.1 40.82,98.57 R142.2 40.32,98.42 R143.1
N$240
  Top 0.406: C153.2 42.55,90.66 Q15.B R144.2
N$241
  Top 0.406: Q15.C 39.64,93.34 C154.1 39.37,94.61 38.42,95.57 R143.2
N$242
  Top 0.406: C176.1 C151.1 43.81,107.05 | 43.81,107.05 39.85,107.05 IC24.2@1 | R145.2 43.81,109.22 43.81,107.05
N$243  (via drill 0.5)
  Top 0.406: IC22.1 21.01,89.48 v19.05,91.44
  Bottom 0.406: v19.05,91.44 19.05,93.98 20.32,95.25 RES3.TP
N$244
  Top 0.406: IC22.9 31.43,87.95 31.75,87.63 33.97,87.63 34.61,88.27 34.61,91.12 R146.2 35.88,91.44 36.83,91.44 36.52,91.12 R147.1 36.88,91.08 C154.2
N$245
  Top 0.406: R148.1 39.69,68.9 C155.2
N$246
  Top 0.406: IC21.1 38.36,74.87 | 38.36,74.87 R148.2 | 38.36,74.87 38.36,75.51 C178.1
N$247
  Top 0.406: R149.2 42.23,86.94 C153.1
N$248  (via drill 0.5)
  Top 0.406: C160.2 R150.1 47.31,86.36 44.13,83.19 v40.64,83.19 | 26.67,80.64 24.13,80.64 22.23,78.74 R127.1 v22.23,81.28 | 26.67,80.64 29.53,80.64 31.11,82.07 31.11,82.55 31.75,83.19 v34.29,83.19 34.92,82.55 R122.1 | IC20.7 26.67,80.64 | IC19.8 12.7,83.82 13.34,83.19 v13.97,83.19
  Bottom 0.406: v34.29,83.19 36.2,85.09 38.73,85.09 v40.64,83.19 | v13.97,83.19 14.61,83.19 15.24,82.55 20.95,82.55 v22.23,81.28
N$249
  Top 0.406: R145.1 R151.2 49.85,108.9 50.8,107.95 C161.1
N$250
  Top 0.406: SG8.+ 9.21,73.66 9.84,73.03 C177.2
N$251
  Top 0.406: R152.1 C177.1 12.88,71.12 Q16.B
N$252
  Top 0.406: C178.2 R153.1
N$253
  Top 0.406: R153.2 38.41,77.78 40.01,79.38 IC21.8
N$254
  Top 0.406: U$4.P$1 59.37,65.22 R154.2
N$255
  Top 0.406: U$4.P$5 50.01,72.24 50.32,72.55 53.17,72.56 53.98,71.75 56.48,71.75 U$4.P$6 57.45,72.06 SP4.+
N$256
  Top 0.406: C147.1 15.88,94.61 15.88,92.71 | 15.88,92.71 15.88,90.81 16.51,90.17 18.73,90.17 20.64,88.27 24.77,88.27 25.08,88.58 IC22.4 | X4.1 15.94,92.78 15.88,92.71
N$257
  Top 0.406: IC22.6 27.62,88.58 25.88,86.84 25.88,86.52 R156.1
N$258
  Top 0.406: R155.1 30.16,87.47 28.89,88.74 IC22.7
N$259
  Top 0.406: S4.3 49.39,111.9 50.16,111.12 53.34,111.12 54.61,109.86 D4.A 55.49,108.58 C180.1 C179.1
N$260
  Top 0.406: S4.2 52.53,113.84 55.24,111.12 57.15,111.12 57.78,110.49 60.33,110.49 60.96,109.86 60.96,104.14 G4.+
N$261  (1 unrouted)
  Top 0.406: C216.2 C215.2 C214.2 C213.2 | C217.2 C218.2 C219.2 C220.2 C211.2 121.28,74.77 | 121.28,74.77 121.29,74.77 C212.2 | 121.28,74.77 121.28,74.3 117.32,74.3 116.36,73.34 116.36,70.96 116.84,70.48 118.23,70.48 U$5.P$4 118.88,70.36 122.56,66.67 125.25,66.67 U$5.P$3
N$262
  Top 0.406: C185.1 114.93,67.63 R162.1
N$263
  Top 0.406: IC27.7 109.86,78.74 110.49,78.11 113.34,78.11 C186.2
N$264
  Top 0.406: IC25.4 85.09,80.64 87,78.74 87.31,78.74 R171.1
N$265
  Top 0.406: R171.2 C191.1
N$266
  Top 0.406: SG9.+ 77.79,84.77 78.74,83.82 C187.2
N$267
  Top 0.406: 80.64,76.69 Q18.B 80.5,76.83 79.69,76.83 79.37,77.16 R157.1 78.42,76.84 78.42,76.83 77.47,78.11 77.47,80.33 78.11,80.97 C187.1
N$268
  Top 0.254: 83.02,76.05 81.6,77.47 80.33,77.47
  Top 0.406: R191.2 83.51,67.63 C188.2 84.46,69.53 85.41,70.48 85.41,71.58 Q20.C 85.24,74.47 R165.2 83.97,74.61 Q18.C 83.02,76.05 | 80.33,77.47 80.01,77.79 80.01,78.74 79.69,79.06 R157.2
N$269
  Top 0.406: 90.8,76.2 R166.2 | C204.1 C203.1 C202.1 C201.1 90.81,73.66 | 90.81,73.66 R166.2 | R165.1 85.72,76.52 R166.2 | R166.2 | 89.53,71.12 R167.1 89.85,70.8 90.81,71.75 90.81,73.66 | 89.53,72.39 90.81,73.66
N$270
  Top 0.406: R169.1 86.68,64.77 | R168.2 86.05,64.78 R169.1 | Q17.B 86.83,64.62 R169.1
N$271
  Top 0.406: C188.1 R169.2
N$272
  Top 0.254: Q17.C 89.22,62.87 88.9,62.55
  Top 0.406: R168.1 88.9,62.55 C189.1 | R167.2 Q17.C
N$273
  Top 0.406: C189.2 91.44,63.5 92.71,64.77 92.71,66.84 R170.1
N$274  (via drill 0.5)
  Top 0.406: IC25.1 v81.28,78.74 | v94.3,70.17 92.08,70.17 R170.2
  Bottom 0.406: v81.28,78.74 83.19,78.74 v94.3,70.17
N$275
  Top 0.406: C190.1 82.87,79.06 82.55,79.38 IC25.2
N$276  (via drill 0.5)
  Top 0.406: v90.17,85.09 87.95,85.09 C191.2
  Bottom 0.406: R164.P$3 105.92,105.53 108.58,102.87 108.58,93.34 100.33,85.09 v90.17,85.09
N$277  (via drill 0.5)
  Top 0.406: v111.76,69.85 111.76,73.34 C184.2 111.44,74.61 111.12,74.93 IC27.3
  Bottom 0.406: R164.P$1 99.81,105.53 101.6,107.31 106.05,107.31 111.76,101.6 v111.76,69.85
N$278
  Top 0.406: C200.1 111.76,67.94 C185.2 112.71,68.26 113.03,68.58 113.03,72.39 113.66,73.02 113.67,73.03 116.52,75.88 116.52,80.01 | 116.52,80.01 116.52,83.5 118.75,85.72 121.28,85.72 121.28,84.77 | 121.28,84.77 123.83,84.77 124.14,84.45 124.14,80.01 C216.1 C215.1 C214.1 C213.1 C212.1 | C211.1 C220.1 C219.1 C218.1 C217.1 118.43,84.46 118.75,84.77 121.28,84.77 | IC27.5 116.46,80.07 116.52,80.01
N$279
  Top 0.406: IC26.3 96.52,79.38 101.28,79.38 R160.2 103.33,79.69 R161.2 105.23,79.52 R159.1
N$280
  Top 0.406: IC26.2 95.25,75.25 C183.2 95.57,72.49 R163.P$3
N$281  (via drill 0.5)
  Top 0.406: IC25.6 83.82,84.45 v84.45,83.82 | 104.46,85.25 96.68,85.25 95.89,84.45 93.34,84.45 92.71,83.82 v92.08,83.82 | C182.2 104.46,86.36 104.46,85.25 | 104.46,85.25 C181.2
  Bottom 0.406: v84.45,83.82 v92.08,83.82
N$282
  Top 0.406: C182.1 105.72,88.9 107,89.22 R172.2
N$283
  Top 0.406: R158.1 100.02,72.69 R163.P$1
N$284  (via drill 0.5)  (1 unrouted)
  Top 0.406: IC28.19 v91.12,97.16 | v85.41,109.86 85.41,110.17 86.04,110.81 86.04,112.08
  Bottom 0.406: SCK4.TP 91.44,97.16 v91.12,97.16 89.22,97.16 85.41,100.97 v85.41,109.86
N$285  (via drill 0.5)  (1 unrouted)
  Top 0.406: R174.1 v87.31,109.85 | v92.08,100.65 92.39,100.33 IC28.18
  Bottom 0.406: MISO4.TP 95.89,97.16 93.98,99.06 92.08,99.06 | 92.08,99.06 88.9,99.06 86.36,101.6 86.36,109.86 v87.31,109.86 | 92.08,99.06 v92.08,100.65
N$286  (via drill 0.5)
  Top 0.406: R175.1 86.04,98.43 86.04,96.84 87.63,95.25 93.03,95.25 93.66,95.89 IC28.17 v93.66,100.33 | v98.42,96.52 98.42,92.08 97.47,91.12 v94.61,91.12
  Bottom 0.406: v93.66,100.33 94.61,100.33 v98.42,96.52 | v94.61,91.12 94.3,91.12 93.34,92.08 MOSI4.TP
N$287
  Top 0.406: R176.1 84.58,97.03 87,94.61 93.98,94.61 94.93,95.57 IC28.16
N$288
  Top 0.406: R177.1 93.66,102.23 96.2,99.69 IC28.15
N$289
  Top 0.406: IC28.14 97.47,100.01 93.15,104.33 R178.1
N$290  (via drill 0.5)
  Top 0.406: R179.1 v88.58,104.78 | v98.74,100.65 IC28.13
  Bottom 0.406: v88.58,104.78 92.71,104.78 94.61,102.87 96.52,102.87 v98.74,100.65
N$291  (1 unrouted)
  Top 0.406: IC28.12 100.01,101.92 99.69,102.23 99.54,102.39 99.06,102.87
N$292
  Top 0.406: R173.2 84.14,111.76 IC29.5
N$293
  Top 0.406: IC29.4 84.46,107.31 R174.2
N$294
  Top 0.406: IC29.10 78.11,99.69 79.38,100.97 84.14,100.97 R175.2
N$295
  Top 0.406: IC29.1 82.23,97.35 R176.2
N$296
  Top 0.406: IC29.2 R177.2
N$297
  Top 0.406: IC29.3 82.87,104.78 84.14,106.05 89.41,106.05 R178.2
N$298
  Top 0.406: IC29.8 75.88,104.78 77.15,103.5 83.82,103.5 R179.2
N$299
  Top 0.406: IC29.7 76.52,107.31 77.79,106.05 83.19,106.05 83.82,106.68 89.85,106.68 90.65,105.89 94.14,105.89 94.3,105.73 94.3,104.62 96.36,102.55 R180.2
N$300  (via drill 0.5)
  Top 0.406: v96.84,87.95 R194.2
  Bottom 0.406: IC29.9 75.88,102.23 76.83,101.28 76.83,98.42 78.74,96.52 78.74,95.25 80.64,93.34 80.64,90.81 83.5,87.95 v96.84,87.95
N$301  (via drill 0.5)
  Top 0.406: R195.2 89.06,86.2 87,88.27 84.45,88.27 v83.19,89.53
  Bottom 0.406: v83.19,89.53 83.19,94.61 77.47,100.33 77.47,108.58 76.2,109.86 IC29.6
N$302
  Top 0.406: C193.1 81.33,92.03 81.92,91.44 82.84,91.44 X5.3 82.91,91.08 84.77,89.22 87.31,89.22 88.9,87.63 93.98,87.63 94.93,88.58 IC28.5
N$303  (via drill 0.5)
  Top 0.406: IC28.20 89.85,100.01 90.17,100.33 v90.17,100.65 C194.2 | v106.68,102.23 107.95,102.23 108.07,102.12 | R185.1 103.5,92.71 v100.33,95.89 | R181.1 109.22,100.97 108.07,102.12 | C195.1 109.86,102.87 | 109.86,102.87 108.82,102.87 108.07,102.12 | 108.07,102.12 | IC30.3 109.86,104.54 109.86,102.87
  Bottom 0.406: v106.68,102.23 102.23,102.23 100.33,100.33 100.33,98.42 | VCC4.TP 97.16,92.71 v100.33,95.89 100.33,98.42 | 100.33,98.42 99.06,98.42 95.25,102.23 90.17,102.23 v90.17,100.65
N$304
  Top 0.406: R183.1 116.2,97.16 114.94,98.42 112.92,98.42 C197.1 109.4,98.57 R181.2 108.9,98.42 R182.1
N$305
  Top 0.406: C198.2 111.12,90.66 Q19.B R183.2
N$306
  Top 0.406: Q19.C 108.22,93.34 C199.1 107.95,94.61 107,95.57 R182.2
N$307
  Top 0.406: C221.1 C196.1 112.39,107.05 | 112.39,107.05 108.43,107.05 IC30.2@1 | R184.2 112.39,109.22 112.39,107.05
N$308  (via drill 0.5)
  Top 0.406: IC28.1 89.59,89.48 v87.63,91.44
  Bottom 0.406: v87.63,91.44 87.63,93.98 88.9,95.25 RES4.TP
N$309
  Top 0.406: IC28.9 100.01,87.95 100.33,87.63 102.55,87.63 103.19,88.27 103.19,91.12 R185.2 104.46,91.44 105.41,91.44 105.09,91.12 R186.1 105.46,91.08 C199.2
N$310
  Top 0.406: R187.1 108.27,68.9 C200.2
N$311
  Top 0.406: IC27.1 106.94,74.87 | 106.94,74.87 R187.2 | 106.94,74.87 106.94,75.51 C223.1
N$312
  Top 0.406: R188.2 110.81,86.94 C198.1
N$313  (via drill 0.5)
  Top 0.406: C205.2 R189.1 115.89,86.36 112.71,83.19 v109.22,83.19 | 95.25,80.64 92.71,80.64 90.81,78.74 R166.1 v90.81,81.28 | 95.25,80.64 98.11,80.64 99.69,82.07 99.69,82.55 100.33,83.19 v102.87,83.19 103.5,82.55 R161.1 | IC26.7 95.25,80.64 | IC25.8 81.28,83.82 81.92,83.19 v82.55,83.19
  Bottom 0.406: v102.87,83.19 104.78,85.09 107.31,85.09 v109.22,83.19 | v82.55,83.19 83.19,83.19 83.82,82.55 89.53,82.55 v90.81,81.28
N$314
  Top 0.406: R184.1 R190.2 118.43,108.9 119.38,107.95 C206.1
N$315
  Top 0.406: SG10.+ 77.79,73.66 78.42,73.03 C222.2
N$316
  Top 0.406: R191.1 C222.1 81.45,71.12 Q20.B
N$317
  Top 0.406: C223.2 R192.1
N$318
  Top 0.406: R192.2 107,77.78 108.58,79.38 IC27.8
N$319
  Top 0.406: U$5.P$1 127.95,65.22 R193.2
N$320
  Top 0.406: U$5.P$5 118.59,72.24 118.9,72.55 121.75,72.56 122.56,71.75 125.06,71.75 U$5.P$6 126.03,72.06 SP5.+
N$321
  Top 0.406: C192.1 84.45,94.61 84.45,92.71 | 84.45,92.71 84.45,90.81 85.09,90.17 87.31,90.17 89.22,88.27 93.34,88.27 93.66,88.58 IC28.4 | X5.1 84.52,92.78 84.45,92.71
N$322
  Top 0.406: IC28.6 96.2,88.58 94.46,86.84 94.46,86.52 R195.1
N$323
  Top 0.406: R194.1 98.74,87.47 97.47,88.74 IC28.7
N$324
  Top 0.406: S5.3 117.97,111.9 118.75,111.12 121.92,111.12 123.19,109.86 D5.A 124.07,108.58 C225.1 C224.1
N$325
  Top 0.406: S5.2 121.11,113.84 123.83,111.12 125.73,111.12 126.36,110.49 128.91,110.49 129.54,109.86 129.54,104.14 G5.+
N$326  (1 unrouted)
  Top 0.406: C261.2 C260.2 C259.2 C258.2 | C262.2 C263.2 C264.2 C265.2 C256.2 189.87,74.77 | 189.87,74.77 C257.2 | 189.87,74.77 189.87,74.3 185.9,74.3 184.94,73.34 184.94,70.96 185.42,70.48 186.81,70.48 U$6.P$4 187.46,70.36 191.13,66.67 193.82,66.67 U$6.P$3
N$327
  Top 0.406: C230.1 183.51,67.63 R201.1
N$328
  Top 0.406: IC33.7 178.44,78.74 179.07,78.11 181.93,78.11 C231.2
N$329
  Top 0.406: IC31.4 153.67,80.64 155.57,78.74 155.89,78.74 R210.1
N$330
  Top 0.406: R210.2 C236.1
N$331
  Top 0.406: SG11.+ 146.37,84.77 147.32,83.82 C232.2
N$332
  Top 0.406: 149.22,76.69 Q22.B 149.07,76.83 148.27,76.83 147.95,77.16 R196.1 147,76.84 147,76.83 146.05,78.11 146.05,80.33 146.69,80.97 C232.1
N$333
  Top 0.254: 151.59,76.05 150.18,77.47 148.91,77.47
  Top 0.406: R230.2 152.09,67.63 C233.2 153.04,69.53 153.99,70.48 153.99,71.58 Q24.C 153.82,74.47 R204.2 152.54,74.61 Q22.C 151.59,76.05 | 148.91,77.47 148.59,77.79 148.59,78.74 148.27,79.06 R196.2
N$334
  Top 0.406: 159.38,76.2 R205.2 | C249.1 C248.1 C247.1 C246.1 159.38,73.66 | 159.38,73.66 R205.2 | R204.1 154.3,76.52 R205.2 | R205.2 | 158.12,71.12 R206.1 158.43,70.8 159.38,71.75 159.38,73.66 | 158.12,72.39 159.38,73.66
N$335
  Top 0.406: R208.1 155.26,64.77 | R207.2 154.62,64.78 R208.1 | Q21.B 155.41,64.62 R208.1
N$336
  Top 0.406: C233.1 R208.2
N$337
  Top 0.254: Q21.C 157.8,62.87 157.48,62.55
  Top 0.406: R207.1 157.48,62.55 C234.1 | R206.2 Q21.C
N$338
  Top 0.406: C234.2 160.02,63.5 161.29,64.77 161.29,66.84 R209.1
N$339  (via drill 0.5)
  Top 0.406: IC31.1 v149.86,78.74 | v162.88,70.17 160.66,70.17 R209.2
  Bottom 0.406: v149.86,78.74 151.76,78.74 v162.88,70.17
N$340
  Top 0.406: C235.1 151.45,79.06 151.13,79.38 IC31.2
N$341  (via drill 0.5)
  Top 0.406: v158.75,85.09 156.53,85.09 C236.2
  Bottom 0.406: R203.P$3 174.5,105.53 177.16,102.87 177.16,93.34 168.91,85.09 v158.75,85.09
N$342  (via drill 0.5)
  Top 0.406: v180.34,69.85 180.34,73.34 C229.2 180.02,74.61 179.71,74.93 IC33.3
  Bottom 0.406: R203.P$1 168.4,105.53 170.18,107.31 174.62,107.31 180.34,101.6 v180.34,69.85
N$343
  Top 0.406: C245.1 180.34,67.94 C230.2 181.29,68.26 181.61,68.58 181.61,72.39 182.24,73.02 182.25,73.03 185.1,75.88 185.1,80.01 | 185.1,80.01 185.1,83.5 187.32,85.72 189.87,85.72 189.87,84.77 | 189.87,84.77 192.41,84.77 192.72,84.45 192.72,80.01 C261.1 C260.1 C259.1 C258.1 C257.1 | C256.1 C265.1 C264.1 C263.1 C262.1 187.01,84.46 187.32,84.77 189.87,84.77 | IC33.5 185.04,80.07 185.1,80.01
N$344
  Top 0.406: IC32.3 165.1,79.38 169.86,79.38 R199.2 171.91,79.69 R200.2 173.81,79.52 R198.1
N$345
  Top 0.406: IC32.2 163.83,75.25 C228.2 164.15,72.49 R202.P$3
N$346  (via drill 0.5)
  Top 0.406: IC31.6 152.4,84.45 v153.03,83.82 | 173.04,85.25 165.26,85.25 164.47,84.45 161.93,84.45 161.29,83.82 v160.66,83.82 | C227.2 173.04,86.36 173.04,85.25 | 173.04,85.25 C226.2
  Bottom 0.406: v153.03,83.82 v160.66,83.82
N$347
  Top 0.406: C227.1 174.31,88.9 175.58,89.22 R211.2
N$348
  Top 0.406: R197.1 168.59,72.69 R202.P$1
N$349  (via drill 0.5)  (1 unrouted)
